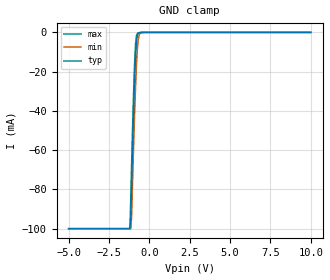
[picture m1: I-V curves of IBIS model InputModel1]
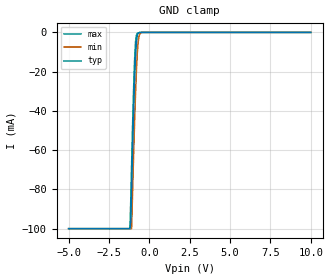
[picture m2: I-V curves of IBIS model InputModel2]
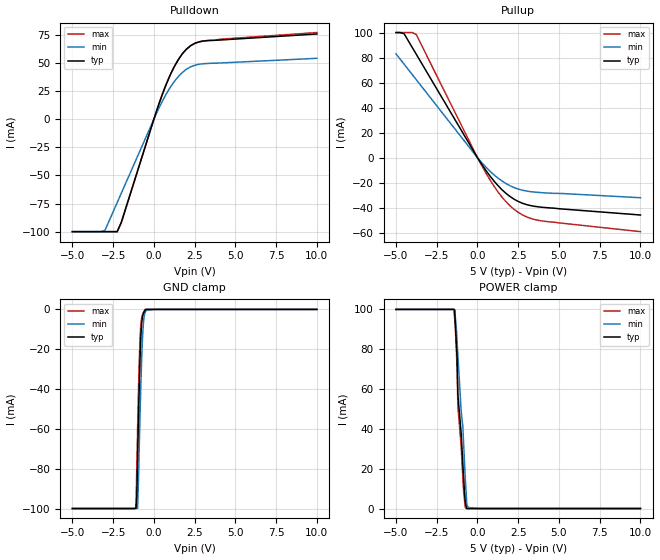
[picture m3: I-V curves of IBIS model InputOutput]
[IBIS Ver]   2.1
[File name]   pa016sc5.ibs   | pa= TSOP, f016sc= abbr chip name, 5= 5V Vcc
[File Rev]   2.00
[Date]   18-April-1996
[Source]   File generated from lab measurements at Intel Corporation
[Notes]   Rev 2.00 All data was replaced by actual measurements
   performed in a lab.
[Disclaimer] INTEL DEVELOPER'S SOFTWARE LICENSE AGREEMENT
| BY USING THIS SOFTWARE, YOU ARE AGREEING TO BE BOUND
| BY THE TERMS OF THIS AGREEMENT.  DO NOT USE THE SOFTWARE
| UNTIL YOU HAVE CAREFULLY READ AND AGREED TO THE FOLLOWING
| TERMS AND CONDITIONS.  IF YOU DO NOT AGREE TO THE TERMS
| OF THIS AGREEMENT, PROMPTLY RETURN THE SOFTWARE PACKAGE
| AND ANY ACCOMPANYING ITEMS.
| IF YOU USE THIS SOFTWARE, YOU WILL BE BOUND BY THE TERMS
| OF THIS AGREEMENT
| LICENSE: Intel Corporation ("Intel") grants you the non-exclusive right
| to use the enclosed software program ("Software").  You will not use,
| copy, modify, rent, sell or transfer the Software or any portion
| thereof, except as provided in this Agreement.
| System OEM Developers may:
| 1.   Copy the Software for support, backup or archival purposes;
| 2.   Install, use, or distribute Intel owned Software in object code
|   only;
| 3.   Modify and/or use Software source code that Intel directly makes
|   available to you as an OEM Developer;
| 4.   Install, use, modify, distribute, and/or make or have made
|   derivatives ("Derivatives") of Intel owned Software under the
|   terms and conditions in this Agreement, ONLY if you are a System
|   OEM Developer and NOT an end-user.
| RESTRICTIONS:
| YOU WILL NOT:
| 1.   Copy the Software, in whole or in part, except as provided for
|   in this Agreement;
| 2.   Decompile or reverse engineer any Software provided in object
|   code format;
| 3.   Distribute any Software or Derivative code to any end-users,
|   unless approved by Intel in a prior writing.
| TRANSFER: You may transfer the Software to another OEM
| Developer if the receiving party agrees to the terms of this
| Agreement at the sole risk of any receiving party.
| OWNERSHIP AND COPYRIGHT OF SOFTWARE:
| Title to the Software and all copies thereof remain with Intel
| or its vendors.  The Software is copyrighted and is protected by
| United States and international copyright laws.  You will not
| remove the copyright notice from the Software.  You agree to
| prevent any unauthorized copying of the Software.
| DERIVATIVE WORK: OEM Developers that make or have made
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[Copyright]   Copyright 1996, Intel Corporation, All Rights Reserved
[Component]   PA28F016SC   | 44-lead PSOP package, 28F016SC
[Manufacturer]  Intel   | Flash File (tm)
|   | operating in 5V Vcc range
[Package]
|The following values apply for the leadframe.
|Variable   typ   min   max
R_pkg   145m   144m   147m
L_pkg   5.25nH   2.00nH   8.50nH
C_pkg   1.09pF   0.68pF   1.50pF
|*****************************Pin Definitions**********************************
[Pin]   signal_name   model_name   R_pin   L_pin   C_pin
  1   VPP   POWER
  2   RP#   InputModel1
  3   A11   InputModel1
  4   A10   InputModel1
  5   A09   InputModel1
  6   A08   InputModel1
  7   A07   InputModel1
  8   A06   InputModel1
  9   A05   InputModel1
 10   A04   InputModel1
 11   NC   InputModel2
 12   NC   InputModel2
 13   A03   InputModel1
 14   A02   InputModel1
 15   A01   InputModel1
 16   A00   InputModel1
 17   DQ0   InputOutput
 18   DQ1   InputOutput
 19   DQ2   InputOutput
 20   DQ3   InputOutput
 21   GND   GND
 22   GND   GND
 23   VCC   POWER
 24   DQ4   InputOutput
 25   DQ5   InputOutput
 26   DQ6   InputOutput
 27   DQ7   InputOutput
 28   RY/BY#   RYBYOutput
 29   OE#   InputModel2
 30   WE#   InputModel2
 31   NC   InputModel2
 32   NC   InputModel2
 33   NC   InputModel2
 34   A20   InputModel1
 35   A19   InputModel1
 36   A18   InputModel1
 37   A17   InputModel1
 38   A16   InputModel1
 39   A15   InputModel1
 40   A14   InputModel1
 41   A13   InputModel1
 42   A12   InputModel1
 43   CE#   InputModel1
 44   VCC   POWER
| Models and submodels in the file (4): InputModel1 (Input), InputModel2 (Input), InputOutput (I/O), RYBYOutput (Output)
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|**************************Input Model 1***************************************
[Model]   InputModel1
Model_type   Input
|   For A[0:20], CE# & RP#.
Vinl = 0.8V
Vinh = 2.0V
| Variable   typ   min   max
C_comp   5.61p   NA   7.6p
[Voltage Range]   5.0V   4.5V   5.5V
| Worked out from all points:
|   GND clamp passes 1 mA (typ) near -0.72 V on its own axis
[GND_clamp]
|Voltage I(typ)   I(min)   I(max)
-5V       -100mA     -100mA     -100mA
-1.2V     -100mA     -100mA     -100mA
-1.15V    -93.74mA   -100mA     -84.05mA
-1.1V     -77.27mA   -93.99mA   -67.55mA
-950mV    -32.75mA   -51.03mA   -23.72mA
-900mV    -20.64mA   -38.23mA   -12.87mA
-850mV    -11.3mA    -27mA      -5.501mA
-800mV    -4.845mA   -17.08mA   -1.805mA
-750mV    -1.73mA    -9.527mA   -608.6uA
-650mV    -262.9uA   -1.924mA   -177.2uA
-500mV    0A         -118.8uA   -20.67uA
10V       0A         0A         0A
[POWER_clamp]
| Input buffer circuits of this product do not intrinsically
| require a [POWER_clamp] definition.  This zero current
| [POWER_clamp] is provided for compatibility with some ibis
| parsers.
|Voltage  I(typ)   I(min)   I(max)
-5V       0A         0A         0A
0V        0A         0A         0A
5V        0A         0A         0A
10V       0A         0A         0A
|**********************Input Model 2************************************
[Model]   InputModel2
Model_type   Input
|   For OE#, WE#, NC Pins
Vinl = 0.8V
Vinh = 2.0V
| Variable   typ   min   max
C_comp   5.61p   NA   7.6p
[Voltage Range]   5.0V   4.5V   5.5V
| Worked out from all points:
|   GND clamp passes 1 mA (typ) near -0.72 V on its own axis
[GND_clamp]
|Voltage I(typ)   I(min)   I(max)
-5V       -100mA     -100mA     -100mA
-1.2V     -100mA     -100mA     -100mA
-1.15V    -96.58mA   -100mA     -85.21mA
-1.1V     -79.47mA   -100mA     -67.78mA
-950mV    -33.28mA   -55.28mA   -22.16mA
-900mV    -20.81mA   -41.71mA   -11.34mA
-850mV    -11.26mA   -29.81mA   -4.466mA
-800mV    -4.78mA    -19.19mA   -1.391mA
-750mV    -1.697mA   -11mA      -498.4uA
-650mV    -257.8uA   -2.403mA   -163.2uA
-500mV    0A         0A         0A
10V       0A         0A         0A
[POWER_clamp]
| Input buffer circuits of this product do not intrinsically
| require a [POWER_clamp] definition.  This zero current
| [POWER_clamp] is provided for compatibility with some ibis
| parsers.
|   Voltage  I(typ)   I(min)   I(max)
-5V       0A         0A         0A
-4.75V    0A         0A         0A
9.75V     0A         0A         0A
10V       0A         0A         0A
|**************************Input Output Model*********************************
[Model]   InputOutput
Model_type   I/O
|   for DQ[0:7]
Vinl = 0.8V
Vinh = 2.0V
| Variable   typ   min   max
C_comp   9.61p   NA   11.6p
[Voltage Range]   5.0V   4.5V   5.5V
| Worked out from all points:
|   slope of the pulldown table from 0 to 0.75 V, typ, clamps not added: 24.4 ohm
|   slope of the pullup table from 0 to 0.75 V, typ, clamps not added: 52.4 ohm
|   GND clamp passes 1 mA (typ) near -0.57 V on its own axis
|   POWER clamp passes 1 mA (typ) near -0.70 V on its own axis
[Pulldown]
| [Pullup] and [Pulldown] IV curves include only the current through
| the channels of output driver transistors when outputs are enabled
| with OE# = VIL.  Although the output driver transistors have np and
| pn diodes inherently created by CMOS IC fabrication between the
| drain and bulk of n-channel and p-channel CMOS transistors,
| the current through these junction diodes is not included in
| [Pullup] or [Pulldown].  Instead that drain/bulk diode current is
| included in the [POWER_clamp] or [GND_clamp] sections, which are
| not dependent on the state of OE# or output data value.
|Voltage  I(typ)   I(min)   I(max)
-5V       -100mA     -100mA     -100mA
-3V       -100mA     -98.8mA    -100mA
-2.25V    -100mA     -74.13mA   -100mA
-2V       -91.7mA    -65.9mA    -92.27mA
0V        0A         0A         -113.8uA
750mV     30.71mA    22.09mA    30.71mA
1.5V      52.86mA    37.86mA    52.86mA
1.75V     58.11mA    41.51mA    58.11mA
2.25V     65.16mA    46.42mA    65.16mA
2.75V     68.55mA    48.65mA    68.55mA
3.25V     69.7mA     49.41mA    69.7mA
10V       75.6mA     54mA       76.9mA
[GND_clamp]
| [POWER_clamp] and [GND_clamp] IV curves describe ESD protection
| circuits PLUS some np and pn diodes which exist between the
| drain and bulk of n-channel and p-channel CMOS transistors.
| These drain/bulk diodes are inherent in CMOS IC fabrication,
| and are visible on the node of the I/O pin at all times.
| Even the drain/bulk diodes of output driver [Pullup] and [Powerdown]
| transistors are included in [POWER_clamp] or [GND_clamp], because
| these diodes contribute to I/O pin current even when the
| chip outputs are tristated by OE# = VIH.
| For example, when V forced on the I/O pin is large, we are
| forward biasing the pn diode at the drain/bulk interface in the
| p-channel pullup transistor.  Similarly, when V forced on the
| I/O pin is sufficiently negative with respect to the substrate
| ground, we are forward biasing the np diode at the drain/bulk
| interface in the n-channel pulldown transistor.  The effects
| of these diodes are included in [POWER_clamp] or [GND_clamp].
|Voltage  I(typ)   I(min)   I(max)
-5V       -100mA     -100mA     -100mA
-1.1V     -99.86mA   -100mA     -99.86mA
-1.05V    -94.45mA   -100mA     -79.81mA
-1V       -74.77mA   -99.86mA   -60.25mA
-950mV    -56.32mA   -86.84mA   -42.05mA
-900mV    -39.3mA    -69.31mA   -26.29mA
-850mV    -25.09mA   -53.11mA   -14.5mA
-800mV    -13.82mA   -37.98mA   -7.336mA
-700mV    -3.661mA   -14.64mA   -2.686mA
-650mV    -2.167mA   -7.6mA     -1.698mA
-550mV    -710.5uA   -1.768mA   0A
10V       0A         0A         0A
[Pullup]
| (Voltages for [Pullup] and [POWER_clamp] are specified with
| negative respect to Vcc.  Reference the IBIS documentation
| for more information regarding Vtable = Vcc - Voutput.
| This method keeps -Vds constant for the values in all three
| columns across a line of the table.
| [Pullup] and [Pulldown] IV curves include only the current through
| the channels of output driver transistors when outputs are enabled
| with OE# = VIL.  Although the output driver transistors have np and
| pn diodes inherently created by CMOS IC fabrication between the
| drain and bulk of n-channel and p-channel CMOS transistors,
| the current through these junction diodes is not included in
| [Pullup] or [Pulldown].  Instead that drain/bulk diode current is
| included in the [POWER_clamp] or [GND_clamp] sections, which are
| not dependent on the state of OE# or output data value.
|Voltage  I(typ)   I(min)   I(max)
-5V       100mA      83.03mA    100mA
-4.5V     99.07mA    74.73mA    100mA
-4V       88.07mA    66.43mA    100mA
-3.75V    82.57mA    62.28mA    98.35mA
0V        0A         0A         0A
500mV     -9.815mA   -7.312mA   -11.84mA
1V        -18.44mA   -13.55mA   -22.46mA
1.5V      -25.56mA   -18.6mA    -31.43mA
2.25V     -33.2mA    -23.9mA    -41.33mA
3V        -37.45mA   -26.63mA   -47.22mA
3.75V     -39.31mA   -27.77mA   -50.08mA
10V       -45.8mA    -32mA      -59.1mA
[POWER_clamp]
| (Voltages for [Pullup] and [POWER_clamp] are specified with
| negative respect to Vcc.  Reference the IBIS documentation
| for more information regarding Vtable = Vcc - Voutput.
| This method keeps -Vds constant for the values in all three
| columns across a line of the table.
| [POWER_clamp] and [GND_clamp] IV curves describe ESD protection
| circuits PLUS some np and pn diodes which exist between the
| drain and bulk of n-channel and p-channel CMOS transistors.
| These drain/bulk diodes are inherent in CMOS IC fabrication,
| and are visible on the node of the I/O pin at all times.
| Even the drain/bulk diodes of output driver [Pullup] and [Powerdown]
| transistors are included in [POWER_clamp] or [GND_clamp], because
| these diodes contribute to I/O pin current even when the
| chip outputs are tristated by OE# = VIH.
| For example, when V forced on the I/O pin is large, we are
| forward biasing the pn diode at the drain/bulk interface in the
| p-channel pullup transistor.  Similarly, when V forced on the
| I/O pin is sufficiently negative with respect to the substrate
| ground, we are forward biasing the np diode at the drain/bulk
| interface in the n-channel pulldown transistor.  The effects
| of these diodes are included in [POWER_clamp] or [GND_clamp].
|Voltage  I(typ)   I(min)   I(max)
-5V       100mA      100mA      100mA
-1.45V    100mA      100mA      100mA
-1.4V     99.62mA    100mA      95.42mA
-1.25V    76.08mA    84.05mA    71.23mA
-1.2V     56.99mA    76.96mA    51.3mA
-1V       37.89mA    49.08mA    31.36mA
-850mV    15.84mA    32.91mA    8.706mA
-700mV    961.7uA    8.664mA    0A
-650mV    0A         1.747mA    0A
-550mV    0A         464.6uA    0A
0V        0A         0A         0A
10V       0A         0A         0A
[Ramp]
| The DQ Ramp information is not provided at this time for the
| device but will be available in the future.  The table below
| is for the compatibility with some IBIS parsers.
| Variable   typ   min   max
 dV/dt_r   0V/0ns   0V/0ns   0V/0ns
 dV/dt_f   0V/0ns   0V/0ns   0V/0ns
